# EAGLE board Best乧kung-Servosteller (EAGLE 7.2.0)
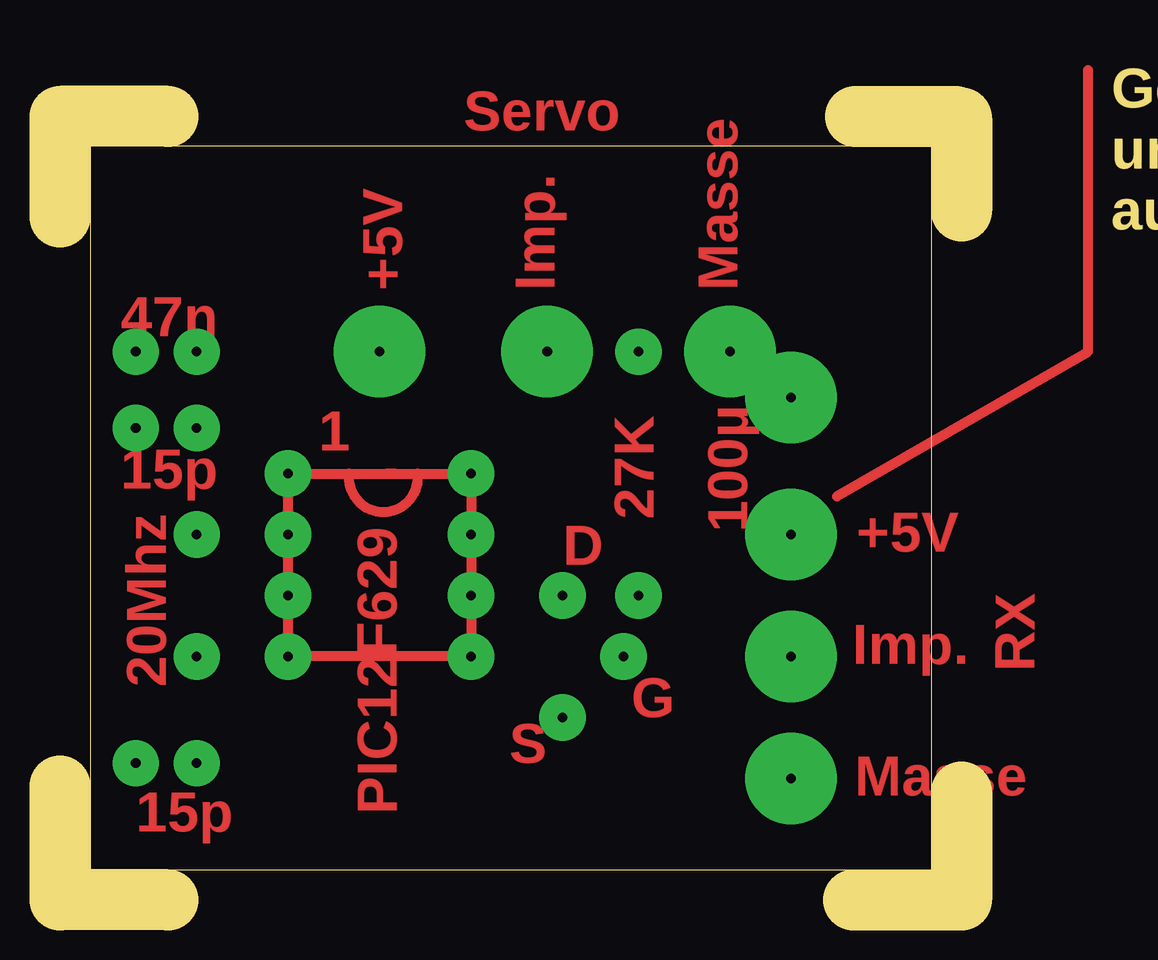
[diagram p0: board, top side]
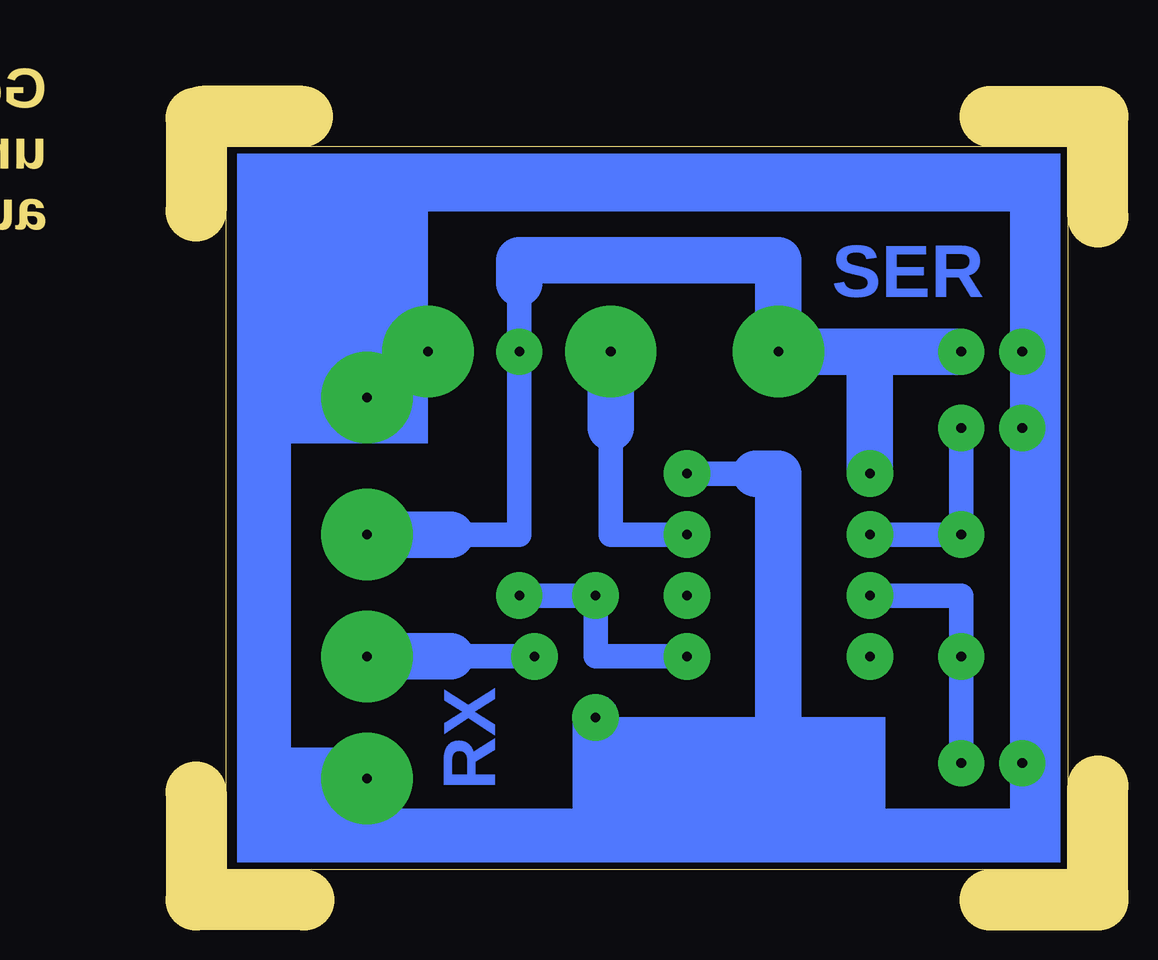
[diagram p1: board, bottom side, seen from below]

Size 37.57 x 32.64 mm. Coordinates in mm from the lower left corner, seen from the top.
Outline: 0,28.46 0,32.64 4.5,32.64
Outline: 0,0.25 0,4.75
Outline: 4.5,0 0,0
Outline: 37.57,32.58 37.57,28.71
Outline: 37.57,4.5 37.57,0 33.07,0
Outline: 33.14,32.64 37.32,32.64
Outline: 1.25,1.25 36.32,1.25 36.32,31.39 1.25,31.39 1.25,1.25
Copper layers (1*16): Top 0.035mm / dielectric 1.5mm / Bottom 0.035mm
Design rules "default": minimum track width 10mil, minimum drill 24mil, track to track 8mil, track to pad 8mil, pad to pad 8mil, via to via 8mil, smd to smd 8mil, copper to edge 40mil, drill to drill 8mil, minimum pad ring 10mil, minimum via ring 8mil, stop-mask expansion 4mil, vias tented up to drill 0mil, thermal gap 10mil

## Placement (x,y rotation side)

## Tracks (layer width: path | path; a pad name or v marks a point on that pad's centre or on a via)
S$1
  Top 0.406: 32.36,16.81 42.84,22.84 42.84,34.59
S$5  (via drill 0.4 pad 1.93, 0.4 pad 3.81)
  Top 0.406: 12.04,17.76 v9.51,17.76 v9.51,10.14 v17.12,10.14 v17.12,17.76 14.9,17.76 | 12.04,17.76 13.63,17.76 | 13.63,17.76 13.95,17.76 | 13.95,17.76 14.9,17.76 | 13.63,17.76 arc-19 13.95,17.76 | 12.04,17.76 arc193 14.9,17.76
  Bottom 1.016: 26.97,15.22 24.11,15.22 v24.11,22.84 24.11,25.7 | v17.12,17.76 14.27,17.76 | 13.31,6.96 13.31,3.16 | 13.31,3.16 3.16,3.16 v3.16,5.7 v3.16,19.66 v3.16,22.84 3.16,29.19 34.91,29.19 34.91,22.84 | 13.31,3.16 20.93,3.16 30.46,3.16 v30.46,5.06 34.91,5.06 34.91,22.84 | 34.91,22.84 v27.92,22.84 | v17.12,10.14 20.93,10.14 v20.93,12.68 v24.11,12.68
  Bottom 1.93: v30.46,15.22 26.97,15.22 | v5.7,22.84 9.51,22.84 | 9.51,22.84 v13.31,22.84 13.31,26.65 24.11,26.65 24.11,25.7 | v9.51,17.76 9.51,22.84 | v20.93,7.6 20.93,3.16 | 13.31,6.96 13.31,17.76 14.27,17.76
  other vias: 30.46,20.93
S$6  (via drill 0.4 pad 1.93, 0.4 pad 3.81)
  Bottom 1.016: v17.12,15.22 20.3,15.22 20.3,19.66
  Bottom 1.93: v20.3,22.84 20.3,19.66
S$7  (via drill 0.4 pad 1.93)
  other vias: 17.12,12.68
S$9  (via drill 0.4 pad 1.93)
  Bottom 1.016: v9.51,15.22 v5.7,15.22 v5.7,19.66
S$11  (via drill 0.4 pad 1.93, 0.4 pad 3.81)
  Bottom 1.016: v23.48,10.14 26.97,10.14 v30.46,10.14
  Bottom 1.93: 26.97,10.14 30.78,10.14
S$13  (via drill 0.4 pad 1.93)
  Bottom 1.016: v5.7,5.7 v5.7,10.14 5.7,12.68 v9.51,12.68
(copper drawn outside any net)
  shapes: Bottom area x10

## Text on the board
Top: Servo | +5V | Imp. | Masse | 47n | 100µ | 1 | 15p | 27K | +5V | PIC12F629 | D | Imp. | 20Mhz | RX | G | Masse | S | 15p
Bottom: SER | RX
Vias: Auf Bestückungsseite gesehen !
Dimension: Gemeinsamer Anschuss +5V (RX) | und für 100µ/16V Elko | auf 1,5mm aufbohren. | Alles mit 0,8mm vorbohren. | Die 6 Anschlüsse für RX und SER auf 1,0mm aufbohren.
tOrigins: 2N7000 | S | D | G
